(* Logix 5000 AddOnInstructionDefinition export L_SHR; software revision 30.00 *)

ADD_ON_INSTRUCTION L_SHR   (* revision 1.0 20170524, vendor Kenneth A. Fischer *)
// LINT bit shift right of the 64-bit argument Inp_A by Inp_B bits with paddding by zeros on the right
// Revision note:
// Rev1.0: 20170524 - Initial Release
VAR_IN_OUT
   Inp_A : LINT; {required}   // 64-bit Integer to be right circular rotated
END_VAR
VAR_INPUT
   Inp_B : INT; {required}   // Number of bits to shift
END_VAR
VAR_IN_OUT
   Out : LINT; {required}   // Result
END_VAR
VAR
   BSR_Cntrl : CONTROL := (LEN := 64);
   ONS : BOOL;
   Source_Bit : BOOL;
   Wrk_InpA : DINT[2];   // Input A as two 32-bit DINTs
END_VAR

ROUTINE Logic   (* ladder *)
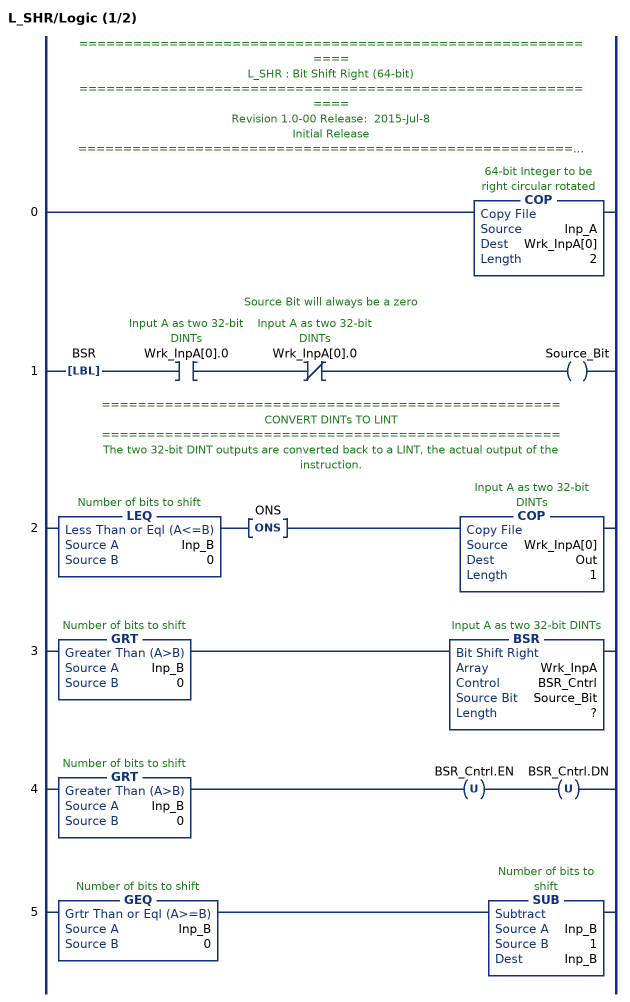
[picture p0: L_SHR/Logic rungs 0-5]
   // ============================================================
   // L_SHR : Bit Shift Right (64-bit)
   // ============================================================
   // Revision 1.0-00 Release:  2015-Jul-8
   // Initial Release
   // ============================================================
   // Performs a right bit shift of the 64-bit argument Inp_A by the
   // number of bits defined in the 16-bit argument Inp_B, with padding by zeros.
   // ===================================================
   // CONVERT LINTs TO DINTs
   // ===================================================
   // These COPies take the input LINTs and break them into pairs of DINTs so we can do math on them.
   // Logix V17 has a LINT data type, but math instructions (and AOI Input and Output Parameters) don't support LINT.
   0: COP(Inp_A,Wrk_InpA[0],2);
   // Source Bit will always be a zero
   1: LBL(BSR)XIC(Wrk_InpA[0].0)XIO(Wrk_InpA[0].0)OTE(Source_Bit);
   // ===================================================
   // CONVERT DINTs TO LINT
   // ===================================================
   // The two 32-bit DINT outputs are converted back to a LINT, the actual output of the instruction.
   2: LEQ(Inp_B,0)ONS(ONS)COP(Wrk_InpA[0],Out,1);
   3: GRT(Inp_B,0)BSR(Wrk_InpA,BSR_Cntrl,Source_Bit,?);
   4: GRT(Inp_B,0)OTU(BSR_Cntrl.EN)OTU(BSR_Cntrl.DN);
   5: GEQ(Inp_B,0)SUB(Inp_B,1,Inp_B);
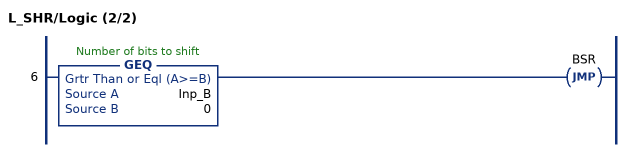
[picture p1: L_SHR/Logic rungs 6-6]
   6: GEQ(Inp_B,0)JMP(BSR);
END_ROUTINE
END_ADD_ON_INSTRUCTION
